| TEXAS INSTRUMENTS INCORPORATED
| Standard Linear and Logic Group
| IBIS Model of SN74AVC16244
| 16-Bit Buffer/Driver With 3-State Outputs
| This file contains package information for the following:
|  TSSOP 48-pin (DGG) package as [Component] AVC16244_DGG
|  TVSOP 48-pin (DGV) package as [Component] AVC16244_DGV
| This device can be powered at the following Vccs:
|  3.3 volt Vcc
|  2.5 volt Vcc
|  1.8 volt Vcc
|  1.5 volt Vcc
|  1.2 volt Vcc
| This file provides unique models under the [Model Selector] for each Vcc.
| For operation at a specific Vcc, select the appropriate model after each
| [Model Selector] keyword.
[IBIS Ver]   3.2
[Comment char]  |_char
[File Name]   sn74avc16244.ibs
[File Rev]   1.2 | x_die
[Date]   March 23, 2006
[Source]   Data created from TI-SPICE simulations at TI-SLL.
[Notes]   The following is an IBIS list for the AVC16244.
   Please contact sllibis@ti.com with questions and
   comments concerning SLL IBIS models.
   - FILE REV HISTORY
   - 1.1 Release IBIS file on 01/27/04
   - 1.2 Release Added GQL package on 3/23/06
   - IBIS 3.2 SYNTAX CANNOT DESCRIBE THE CHARACTERISTICS OF
   ANY OUTPUT STRUCTURES THAT DYNAMICALLY CHANGES THE
   IMPEDANCES DURING THE TRANSITION. THIS DEVICE USE SIMILAR
   OUTPUT STRUCTURE AND THEREFORE THE SIMULATION RESULTS
   MAY NOT BE ACCURATE. TI RECOMMENDS THE USE OF SPICE
   SIMULATION WHEN SIMULATION ACCURACY IS IMPORTANT.
   - Power clamp data deleted as there is no power-clamp diode.
[Disclaimer] Property of Texas Instruments Incorporated.  Unauthorized
   reproduction and/or distribution is strictly prohibited.
   This product is protected under copyright law.
   Created  2004, (C) Copyright  2004, Texas Instruments
   Incorporated, All Rights Reserved
   UNLESS THERE IS A SIGNED, WRITTEN AGREEMENT TO THE
   CONTRARY, TEXAS INSTRUMENTS (TI) IS PROVIDING THE IBIS
   MODELS  AND WITHOUT ANY WARRANTY, EXPRESSED OR
   IMPLIED.  TI assumes no liability for:
   1) the accuracy of the IBIS models provided to your
   company;
   2) the proper functioning of these IBIS Models in your
   design or for any resulting applications; or
   3) infringement of patents, copyrights or intellectual
   property rights resulting from your use of these IBIS
   models.
   TI provides IBIS Models as a service to our customers.
   You and your company shall not distribute, sell or give
   these models to anyone else without prior written
   permission from TI.
   TI reserves the right to make changes to our products or
   to discontinue any semiconductor product or service
   without notice, and advises our customers to obtain the
   latest version of relevant information to verify, before
   placing orders, that the information being relied on is
   current.
   Please be aware that your receipt and use of the IBIS
   information provided shall serve as acceptance of these
   terms and conditions.  If you do not accept these terms,
   you should return or destroy the IBIS models and any
   other accompanying information immediately.
| Component AVC16244_DGG 48-pin TSSOP
[Component]   AVC16244_DGG
[Manufacturer]   Texas Instruments, Inc.
[Package]
|   typ   min   max
R_pkg   4.400e-02   3.800e-02   5.100e-02
L_pkg   3.019e-09   2.486e-09   4.099e-09
C_pkg   5.070e-13   3.340e-13   8.090e-13
[Pin]   signal_name   model_name   R_pin   L_pin   C_pin
1   1OE   AVC16244_IN   4.100e-02   4.017e-09   7.590e-13
2   1Y1   AVC16244_OUT   4.200e-02   3.737e-09   7.920e-13
3   1Y2   AVC16244_OUT   4.200e-02   3.480e-09   6.610e-13
4   GND   GND   3.800e-02   3.131e-09   5.750e-13
5   1Y3   AVC16244_OUT   4.700e-02   3.122e-09   5.660e-13
6   1Y4   AVC16244_OUT   4.300e-02   2.948e-09   5.040e-13
7   VCC   POWER   4.500e-02   2.845e-09   3.970e-13
8   2Y1   AVC16244_OUT   4.900e-02   2.835e-09   3.940e-13
9   2Y2   AVC16244_OUT   4.800e-02   2.715e-09   3.780e-13
10   GND   GND   5.000e-02   2.664e-09   3.630e-13
11   2Y3   AVC16244_OUT   5.000e-02   2.585e-09   3.480e-13
12   2Y4   AVC16244_OUT   4.900e-02   2.550e-09   3.370e-13
13   3Y1   AVC16244_OUT   4.900e-02   2.541e-09   3.360e-13
14   3Y2   AVC16244_OUT   5.000e-02   2.574e-09   3.480e-13
15   GND   GND   4.900e-02   2.618e-09   3.590e-13
16   3Y3   AVC16244_OUT   4.600e-02   2.671e-09   3.750e-13
17   3Y4   AVC16244_OUT   4.500e-02   2.754e-09   3.890e-13
18   VCC   POWER   4.400e-02   2.823e-09   4.500e-13
19   4Y1   AVC16244_OUT   4.200e-02   2.968e-09   5.030e-13
20   4Y2   AVC16244_OUT   5.100e-02   3.108e-09   5.350e-13
21   GND   GND   4.200e-02   3.175e-09   5.870e-13
22   4Y3   AVC16244_OUT   4.100e-02   3.449e-09   6.780e-13
23   4Y4   AVC16244_OUT   4.400e-02   3.766e-09   8.040e-13
24   4OE   AVC16244_IN   4.300e-02   4.065e-09   7.610e-13
25   3OE   AVC16244_IN   4.100e-02   3.994e-09   7.570e-13
26   4A4   AVC16244_IN   3.900e-02   3.649e-09   7.890e-13
27   4A3   AVC16244_IN   3.800e-02   3.362e-09   6.600e-13
28   GND   GND   3.800e-02   3.082e-09   5.740e-13
29   4A2   AVC16244_IN   4.400e-02   2.990e-09   5.220e-13
30   4A1   AVC16244_IN   4.100e-02   2.917e-09   4.950e-13
31   VCC   POWER   4.300e-02   2.820e-09   4.480e-13
32   3A4   AVC16244_IN   4.300e-02   2.699e-09   3.850e-13
33   3A3   AVC16244_IN   4.500e-02   2.628e-09   3.720e-13
34   GND   GND   4.600e-02   2.556e-09   3.560e-13
35   3A2   AVC16244_IN   4.600e-02   2.495e-09   3.440e-13
36   3A1   AVC16244_IN   4.700e-02   2.487e-09   3.340e-13
37   2A4   AVC16244_IN   4.700e-02   2.490e-09   3.350e-13
38   2A3   AVC16244_IN   4.600e-02   2.486e-09   3.430e-13
39   GND   GND   4.500e-02   2.566e-09   3.560e-13
40   2A2   AVC16244_IN   4.400e-02   2.639e-09   3.740e-13
41   2A1   AVC16244_IN   4.300e-02   2.701e-09   3.860e-13
42   VCC   POWER   4.300e-02   2.817e-09   4.500e-13
43   1A4   AVC16244_IN   4.100e-02   2.935e-09   5.010e-13
44   1A3   AVC16244_IN   4.700e-02   3.035e-09   5.290e-13
45   GND   GND   4.300e-02   3.171e-09   5.890e-13
46   1A2   AVC16244_IN   4.000e-02   3.415e-09   6.820e-13
47   1A1   AVC16244_IN   4.300e-02   3.741e-09   8.090e-13
48   2OE   AVC16244_IN   4.400e-02   4.099e-09   7.640e-13
| Component AVC16244_DGV 48-pin TVSOP
[Component]   AVC16244_DGV
[Manufacturer]   Texas Instruments, Inc.
[Package]
|   typ   min   max
R_pkg   7.000e-02   4.900e-02   8.500e-02
L_pkg   3.013e-09   2.743e-09   3.408e-09
C_pkg   3.710e-13   2.940e-13   5.110e-13
[Pin]   signal_name   model_name   R_pin   L_pin   C_pin
1   1OE   AVC16244_IN   4.900e-02   3.393e-09   4.970e-13
2   1Y1   AVC16244_OUT   6.000e-02   3.250e-09   5.020e-13
3   1Y2   AVC16244_OUT   7.700e-02   3.310e-09   4.510e-13
4   GND   GND   8.500e-02   3.299e-09   4.040e-13
5   1Y3   AVC16244_OUT   8.300e-02   3.136e-09   3.600e-13
6   1Y4   AVC16244_OUT   7.700e-02   3.019e-09   3.630e-13
7   VCC   POWER   6.500e-02   2.882e-09   3.490e-13
8   2Y1   AVC16244_OUT   6.600e-02   2.829e-09   3.140e-13
9   2Y2   AVC16244_OUT   6.700e-02   2.796e-09   3.140e-13
10   GND   GND   6.900e-02   2.754e-09   3.080e-13
11   2Y3   AVC16244_OUT   7.000e-02   2.753e-09   3.010e-13
12   2Y4   AVC16244_OUT   7.100e-02   2.745e-09   2.940e-13
13   3Y1   AVC16244_OUT   7.000e-02   2.744e-09   2.940e-13
14   3Y2   AVC16244_OUT   7.000e-02   2.754e-09   3.010e-13
15   GND   GND   6.900e-02   2.754e-09   3.080e-13
16   3Y3   AVC16244_OUT   6.700e-02   2.796e-09   3.140e-13
17   3Y4   AVC16244_OUT   6.600e-02   2.829e-09   3.140e-13
18   VCC   POWER   6.500e-02   2.883e-09   3.500e-13
19   4Y1   AVC16244_OUT   7.500e-02   3.014e-09   3.630e-13
20   4Y2   AVC16244_OUT   8.000e-02   3.128e-09   3.580e-13
21   GND   GND   8.400e-02   3.295e-09   4.030e-13
22   4Y3   AVC16244_OUT   7.800e-02   3.311e-09   4.520e-13
23   4Y4   AVC16244_OUT   6.200e-02   3.259e-09   5.010e-13
24   4OE   AVC16244_IN   5.200e-02   3.404e-09   4.960e-13
25   3OE   AVC16244_IN   5.300e-02   3.397e-09   5.050e-13
26   4A4   AVC16244_IN   6.200e-02   3.249e-09   5.110e-13
27   4A3   AVC16244_IN   7.700e-02   3.308e-09   4.530e-13
28   GND   GND   8.200e-02   3.289e-09   4.030e-13
29   4A2   AVC16244_IN   7.800e-02   3.121e-09   3.590e-13
30   4A1   AVC16244_IN   7.400e-02   3.010e-09   3.630e-13
31   VCC   POWER   6.500e-02   2.883e-09   3.490e-13
32   3A4   AVC16244_IN   6.700e-02   2.829e-09   3.140e-13
33   3A3   AVC16244_IN   6.700e-02   2.795e-09   3.140e-13
34   GND   GND   6.900e-02   2.753e-09   3.070e-13
35   3A2   AVC16244_IN   7.000e-02   2.753e-09   3.010e-13
36   3A1   AVC16244_IN   7.000e-02   2.743e-09   2.940e-13
37   2A4   AVC16244_IN   7.000e-02   2.743e-09   2.940e-13
38   2A3   AVC16244_IN   7.000e-02   2.753e-09   3.010e-13
39   GND   GND   6.900e-02   2.754e-09   3.070e-13
40   2A2   AVC16244_IN   6.800e-02   2.797e-09   3.140e-13
41   2A1   AVC16244_IN   6.700e-02   2.830e-09   3.140e-13
42   VCC   POWER   6.400e-02   2.880e-09   3.490e-13
43   1A4   AVC16244_IN   7.200e-02   3.004e-09   3.620e-13
44   1A3   AVC16244_IN   7.800e-02   3.121e-09   3.590e-13
45   GND   GND   8.400e-02   3.296e-09   4.030e-13
46   1A2   AVC16244_IN   7.700e-02   3.308e-09   4.510e-13
47   1A1   AVC16244_IN   6.200e-02   3.258e-09   4.990e-13
48   2OE   AVC16244_IN   5.300e-02   3.408e-09   4.940e-13
| Component AVC16244_GQL 56-pin jrBGA
[Component]   AVC16244_GQL
[Manufacturer]   Texas Instruments, Inc.
[Package]
|   typ   min   max
R_pkg   6.500e-02   3.500e-02   9.700e-02
L_pkg   1.952e-09   1.000e-09   3.191e-09
C_pkg   2.830e-13   1.620e-13   4.340e-13
[Pin]   signal_name   model_name   R_pin   L_pin   C_pin
A1   1OE   AVC16244_IN   3.600e-02   1.004e-09   1.760e-13
B2   1Y1   AVC16244_OUT   4.000e-02   1.191e-09   1.860e-13
B1   1Y2   AVC16244_OUT   4.700e-02   1.411e-09   2.090e-13
B3   GND   GND   9.700e-02   3.191e-09   4.340e-13
C2   1Y3   AVC16244_OUT   7.400e-02   2.213e-09   3.290e-13
C1   1Y4   AVC16244_OUT   6.000e-02   1.712e-09   2.430e-13
C3   VCC   POWER   8.500e-02   2.691e-09   3.680e-13
D2   2Y1   AVC16244_OUT   7.400e-02   2.160e-09   3.150e-13
D1   2Y2   AVC16244_OUT   6.000e-02   1.666e-09   2.470e-13
D3   GND   GND   7.400e-02   2.121e-09   3.130e-13
E2   2Y3   AVC16244_OUT   9.100e-02   2.924e-09   3.970e-13
E1   2Y4   AVC16244_OUT   6.000e-02   1.619e-09   2.450e-13
F1   3Y1   AVC16244_OUT   6.900e-02   2.031e-09   2.880e-13
F2   3Y2   AVC16244_OUT   6.000e-02   1.583e-09   2.200e-13
G3   GND   GND   6.000e-02   1.578e-09   2.200e-13
G1   3Y3   AVC16244_OUT   6.900e-02   2.017e-09   2.860e-13
G2   3Y4   AVC16244_OUT   6.000e-02   1.594e-09   2.410e-13
H3   VCC   POWER   9.200e-02   2.917e-09   3.970e-13
H1   4Y1   AVC16244_OUT   7.500e-02   2.114e-09   3.150e-13
H2   4Y2   AVC16244_OUT   6.000e-02   1.632e-09   2.470e-13
J3   GND   GND   7.000e-02   2.074e-09   3.070e-13
J1   4Y3   AVC16244_OUT   8.600e-02   2.664e-09   3.650e-13
J2   4Y4   AVC16244_OUT   6.000e-02   1.689e-09   2.490e-13
K1   4OE   AVC16244_IN   6.600e-02   2.152e-09   3.320e-13
K6   3OE   AVC16244_IN   8.700e-02   3.118e-09   4.230e-13
J5   4A4   AVC16244_IN   3.800e-02   1.303e-09   2.000e-13
J6   4A3   AVC16244_IN   3.500e-02   1.176e-09   1.830e-13
J4   GND   GND   3.500e-02   1.007e-09   1.620e-13
H5   4A2   AVC16244_IN   3.500e-02   1.000e-09   1.620e-13
H6   4A1   AVC16244_IN   3.500e-02   1.154e-09   1.800e-13
H4   VCC   POWER   4.100e-02   1.352e-09   2.040e-13
G5   3A4   AVC16244_IN   8.800e-02   3.137e-09   4.300e-13
G6   3A3   AVC16244_IN   7.400e-02   2.218e-09   3.340e-13
G4   GND   GND   6.000e-02   1.683e-09   2.500e-13
F5   3A2   AVC16244_IN   8.500e-02   2.658e-09   3.720e-13
F6   3A1   AVC16244_IN   7.500e-02   2.149e-09   3.210e-13
E6   2A4   AVC16244_IN   6.000e-02   1.627e-09   2.480e-13
E5   2A3   AVC16244_IN   7.500e-02   2.113e-09   3.140e-13
D4   GND   GND   9.200e-02   2.922e-09   3.960e-13
D6   2A2   AVC16244_IN   6.000e-02   1.594e-09   2.420e-13
D5   2A1   AVC16244_IN   6.900e-02   2.016e-09   2.880e-13
C4   VCC   POWER   6.000e-02   1.580e-09   2.210e-13
C6   1A4   AVC16244_IN   6.000e-02   1.582e-09   2.200e-13
C5   1A3   AVC16244_IN   6.900e-02   2.026e-09   2.890e-13
B4   GND   GND   6.000e-02   1.610e-09   2.450e-13
B6   1A2   AVC16244_IN   9.200e-02   2.933e-09   3.960e-13
B5   1A1   AVC16244_IN   7.500e-02   2.126e-09   3.110e-13
A6   2OE   AVC16244_IN   6.000e-02   1.641e-09   2.450e-13
| Model AVC16244_IN
[Model Selector]   AVC16244_IN
AVC16244_IN_33   3.3 volt Vcc
AVC16244_IN_25   2.5 volt Vcc
AVC16244_IN_18   1.8 volt Vcc
AVC16244_IN_15   1.5 volt Vcc
AVC16244_IN_12   1.2 volt Vcc
| Model AVC16244_OUT
[Model Selector]   AVC16244_OUT
AVC16244_OUT_33   3.3 volt Vcc
AVC16244_OUT_25   2.5 volt Vcc
AVC16244_OUT_18   1.8 volt Vcc
AVC16244_OUT_15   1.5 volt Vcc
AVC16244_OUT_12   1.2 volt Vcc
| Models and submodels in the file (10): AVC16244_IN_33 (Input), AVC16244_IN_25 (Input), AVC16244_IN_18 (Input), AVC16244_IN_15 (Input), AVC16244_IN_12 (Input), AVC16244_OUT_33 (3-state), AVC16244_OUT_25 (3-state), AVC16244_OUT_18 (3-state), AVC16244_OUT_15 (3-state), AVC16244_OUT_12 (3-state)
